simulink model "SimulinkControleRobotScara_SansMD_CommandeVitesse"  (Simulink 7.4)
settings: Solver=ode45  StartTime=0.0  StopTime=T  FixedStep=0.1  MaxStep=0.1  MinStep=0.01  RelTol=0.1  AbsTol=0.01
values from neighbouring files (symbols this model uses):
  theta1 = theta1_last+n*Deltatheta1    [GestionGUI.m]    (also in ModeleGeometriqueDirect.m = Theta(1); ModeleGeometriqueInverse.m = alpha - beta; SimulationRobotSCARA.m = 1.57079632679)
  theta2 = theta2_last+n*Deltatheta2    [GestionGUI.m]    (also in ModeleGeometriqueDirect.m = Theta(2); ModeleGeometriqueInverse.m = acos((x^2+y^2-l1^2-l2^2)/(2*l1*l2)); SimulationRobotSCARA.m = 1.57079632679)
libraries: simulink x2

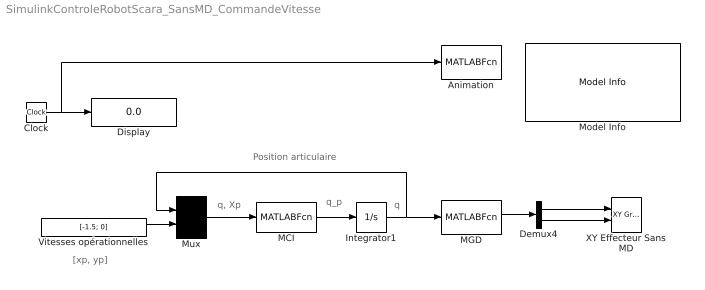
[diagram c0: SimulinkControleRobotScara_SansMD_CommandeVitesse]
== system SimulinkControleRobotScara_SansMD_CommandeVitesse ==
  note: Position articulaire
  note: q_p
  note: q
  note: q, Xp
  note: [xp, yp]
  Animation : MATLABFcn  Tag=Affichage  Description=Affichage  MATLABFcn=SetAffichage  OutputDimensions=0
  Clock : Clock
  Demux4 : Demux  Outputs=2
  Display : Display
  Integrator1 : Integrator  InitialCondition=[theta1 theta2]
  MCI : MATLABFcn  MATLABFcn=MCI  OutputDimensions=2
  MGD : MATLABFcn  MATLABFcn=ModeleGeometriqueDirect  OutputDimensions=2
  Model Info : simulink/Model-Wide Utilities/Model Info  SystemSampleTime=-1  InitialBlockCM=None  BlockCM=None  Frame=on  DisplayStringWithTags=|  HorizontalTextAlignment=Left  LeftAlignmentValue=0.02  SourceBlockDiagram=SimulinkControleRobotScara_SansMD_CommandeVitesse  TagMaxNumber=20
      | Commande en vitesse 
      | du robot SCARA 2D RR
      | 
      | Lounis Adouane
      | Polytech'Clermont-Ferrand
  Mux : Mux  Inputs=2
  Vitesses opérationnelles : Constant  Value=[-1.5; 0]  OutDataType=sfix(16)  OutScaling=2^0
  XY Effecteur Sans MD : simulink/Sinks/XY Graph  SystemSampleTime=-1  xmin=-20  xmax=20  ymin=-3  ymax=20  st=-1
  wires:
  Clock/1 -> Display/1, Animation/1
  Integrator1/1 -> Mux/1, MGD/1
  Vitesses opérationnelles/1 -> Mux/2
  MCI/1 -> Integrator1/1
  Mux/1 -> MCI/1
  Demux4/1 -> XY Effecteur Sans MD/1
  Demux4/2 -> XY Effecteur Sans MD/2
  MGD/1 -> Demux4/1
